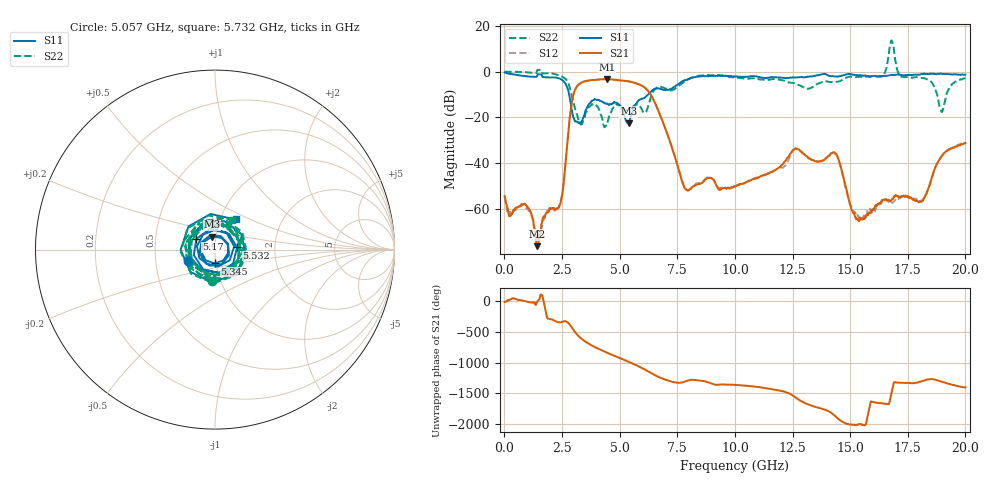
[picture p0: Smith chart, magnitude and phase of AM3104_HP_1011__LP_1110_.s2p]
!Created with skrf (http://scikit-rf.org).
# Hz S RI R 50.0
!freq ReS11 ImS11 ReS21 ImS21 ReS12 ImS12 ReS22 ImS22
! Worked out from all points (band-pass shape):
!   1601 points, 10 MHz to 20 GHz, reference 50 ohm
!   highest |S21| = -3.29 dB at 4.458 GHz (marker M1); lowest = -76.3 dB at 1.434 GHz (marker M2)
!   |S21| within 3 dB of the highest: 3.164 GHz to 5.989 GHz (2.825 GHz wide, 61.7 % of centre)
!   lowest |S11| = -22.6 dB at 5.395 GHz (marker M3), VSWR 1.16, Z = 47.9 + j6.93 ohm
!   |S11| at or under -10 dB: 2.809 GHz to 6.233 GHz (3.424 GHz wide, 75.7 % of centre)
!   |S22| runs from -24.4 to 13.6 dB; largest |S21 - S12| = 0.076
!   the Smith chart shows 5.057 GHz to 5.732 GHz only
!   S11 on the Smith chart (normalised r, x): 5.057 GHz: 0.74, -0.10; 5.17 GHz: 0.81, +0.10; 5.345 GHz: 0.99, -0.15; 5.532 GHz: 1.28, +0.03; 5.732 GHz: 1.18, +0.41
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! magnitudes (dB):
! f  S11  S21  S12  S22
! 10 MHz  -0.4  -54.5  -54.4  0.0
! 1.434 GHz  -1.5  -76.3  -74.1  0.7
! 2.421 GHz  -3.1  -57.9  -57.5  -1.8
! 2.934 GHz  -17.3  -13.0  -13.0  -10.9
! 3.346 GHz  -22.0  -4.8  -4.9  -23.1
! 4.458 GHz  -14.0  -3.3  -3.3  -23.4
! 5.057 GHz  -15.8  -3.8  -3.9  -15.2
! 5.17 GHz  -18.4  -3.9  -4.0  -16.2
! 5.345 GHz  -22.3  -4.2  -4.2  -16.9
! 5.395 GHz  -22.6  -4.3  -4.3  -16.9
! 5.532 GHz  -18.2  -4.6  -4.6  -15.7
! 5.732 GHz  -13.8  -5.2  -5.2  -14.3
! 6.682 GHz  -7.3  -17.1  -17.2  -6.6
! 7.881 GHz  -3.7  -51.5  -51.4  -3.9
! 10.01 GHz  -2.2  -50.3  -50.3  -2.7
! 13.34 GHz  -2.2  -38.7  -38.7  -6.9
! 14.38 GHz  -2.1  -35.9  -36.2  -4.5
! 15.3 GHz  -1.5  -64.5  -62.8  -2.3
! 16.68 GHz  -1.6  -56.4  -57.2  7.3
! 18.11 GHz  -1.0  -56.7  -56.8  -2.8
! 18.96 GHz  -1.0  -37.0  -37.2  -17.5
! 20 GHz  -1.3  -31.3  -30.8  -2.9
